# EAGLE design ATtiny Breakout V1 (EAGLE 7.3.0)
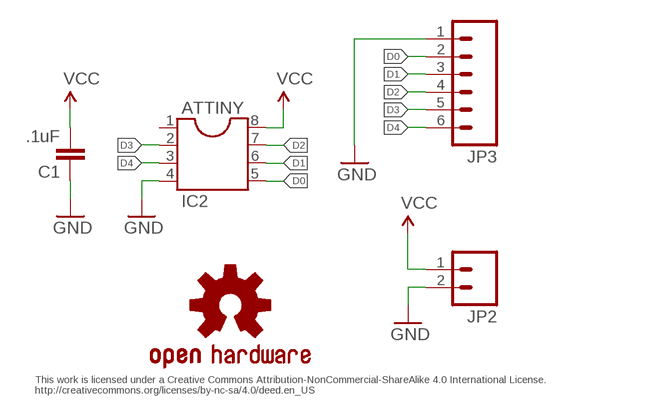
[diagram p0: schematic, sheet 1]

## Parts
ATTINY  IC2  DIL8  [DIL08]
C1  .1uF  CAP0805  [0805]
JP2  M02PTH  [1X02]
JP3  M06SILK_FEMALE_PTH  [1X06]
LOGO2  OSHW-LOGOS  [OSHW-LOGO-S]

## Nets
D0: ATTINY.5 JP3.2
D1: ATTINY.6 JP3.3
D2: ATTINY.7 JP3.4
D3: ATTINY.2 JP3.5
D4: ATTINY.3 JP3.6
GND: ATTINY.4 C1.1 JP2.2 JP3.1
VCC: ATTINY.8 C1.2 JP2.1
Unconnected: ATTINY.1

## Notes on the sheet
- This work is licensed under a Creative Commons Attribution-NonCommercial-ShareAlike 4.0 International License.
  http://creativecommons.org/licenses/by-nc-sa/4.0/deed.en_US

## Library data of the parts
ATTINY = ic-package:DIL8: Dual In Line / Socket
C1 = SparkFun-Passives:CAP: Capacitor
JP2 = SparkFun-Connectors:M02: Standard 2-pin 0.1" header. Use with
JP3 = SparkFun-Connectors:M06: Header 6 Standard 6-pin 0.1" header. Use with straight break away headers (SKU : PRT-00116), right angle break away headers (PRT-00553), swiss pins (PRT-00743), machine pins (PRT-00117), and female headers (PRT-00115). Molex polarized connector foot print use with SKU : PRT-08094 with associated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; PROD_ID: CONN-08437
LOGO2 = SparkFun-Aesthetics:OSHW-LOGO: Open Source Hardware Logo

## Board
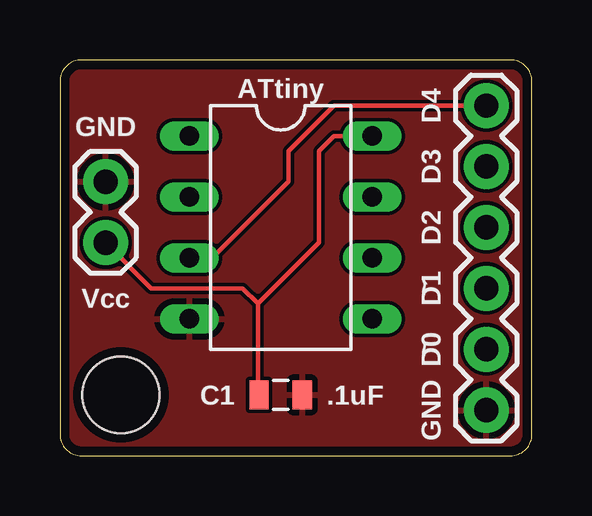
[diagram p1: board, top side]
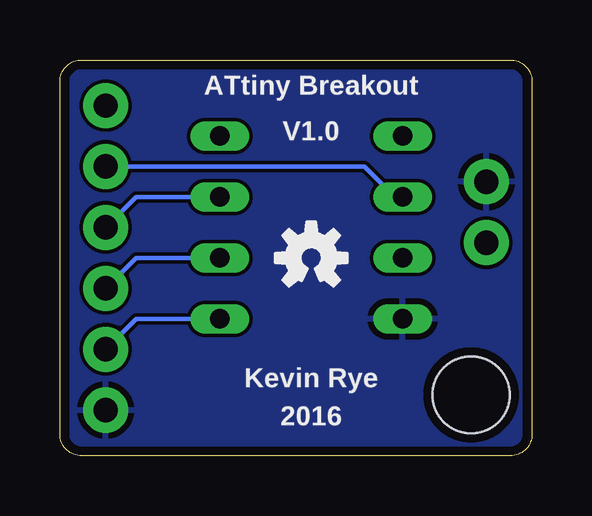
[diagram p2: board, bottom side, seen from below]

Size 19.68 x 16.51 mm. Coordinates in mm from the lower left corner, seen from the top.
Outline: 19.68,0.9 19.68,15.61 arc90 18.79,16.51 0.9,16.51 arc90 0,15.61 0,0.9 arc90 0.9,0 18.79,0 arc90 19.68,0.9
Copper layers (1*16): Top 0.0356mm / dielectric 1.5011mm / Bottom 0.0356mm
Design rules "oshpark-2layer": minimum track width 6mil, minimum drill 13mil, track to track 6mil, track to pad 6mil, pad to pad 6mil, via to via 6mil, smd to smd 6mil, copper to edge 15mil, drill to drill 6mil, minimum pad ring 7mil, minimum via ring 7mil, stop-mask expansion 2.5mil, vias tented up to drill 0mil, thermal gap 10mil
Holes 3.2 mm at 2.54,2.54

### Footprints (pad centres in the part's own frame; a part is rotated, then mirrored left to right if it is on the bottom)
DIL08 = drill 0.813 long: 1 -3.81,-3.81; 2 -1.27,-3.81; 3 1.27,-3.81; 4 3.81,-3.81; 5 3.81,3.81; 6 1.27,3.81; 7 -1.27,3.81; 8 -3.81,3.81
0805 = smd 0.8 x 1.2: 1 -0.9,0; 2 0.9,0
1X02 = drill 1.016 pad 1.88: 1 0,0; 2 2.54,0
1X06 = drill 1.016 pad 1.88: 1 0,0; 2 2.54,0; 3 5.08,0; 4 7.62,0; 5 10.16,0; 6 12.7,0

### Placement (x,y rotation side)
ATTINY  9.21,9.53 270 top
C1  9.21,2.54 180 top
JP2  1.91,8.89 90 top
JP3  17.78,1.91 90 top
LOGO2  9.21,8.26 0 bottom

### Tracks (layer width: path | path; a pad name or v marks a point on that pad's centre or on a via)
D0
  Bottom 0.178: ATTINY.5 16.51,5.71 JP3.2
D1
  Bottom 0.178: ATTINY.6 16.51,8.26 JP3.3
D2
  Bottom 0.178: ATTINY.7 16.51,10.79 JP3.4
D3
  Bottom 0.178: ATTINY.2 5.71,10.79 6.99,12.06 JP3.5
D4
  Top 0.178: ATTINY.3 6.35,8.26 9.53,11.43 9.53,12.7 11.43,14.61 JP3.6
GND
  pour Bottom: -1.27,17.78 20.95,17.78 20.95,-1.27 -1.27,-1.27
  pour Top: -0.64,17.14 20.32,17.14 20.32,-0.64 -0.64,-0.64
VCC
  Top 0.178: JP2.1 3.81,6.99 7.62,6.99 8.26,6.35 | 8.26,6.35 8.26,2.59 C1.2 | ATTINY.8 11.43,13.34 10.79,12.7 10.79,8.89 8.26,6.35

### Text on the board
Unrouted: This work is licensed under a Creative Commons Attribution-NonCommercial-ShareAlike 4.0 International License. / http://creativecommons.org/licenses/by-nc-sa/4.0/deed.en_US
tNames: ATtiny | D4 | GND | D3 | D2 | Vcc | ~ | D1 | ~ | D0 | GND
bNames: ATtiny Breakout | V1.0 | Kevin Rye | 2016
